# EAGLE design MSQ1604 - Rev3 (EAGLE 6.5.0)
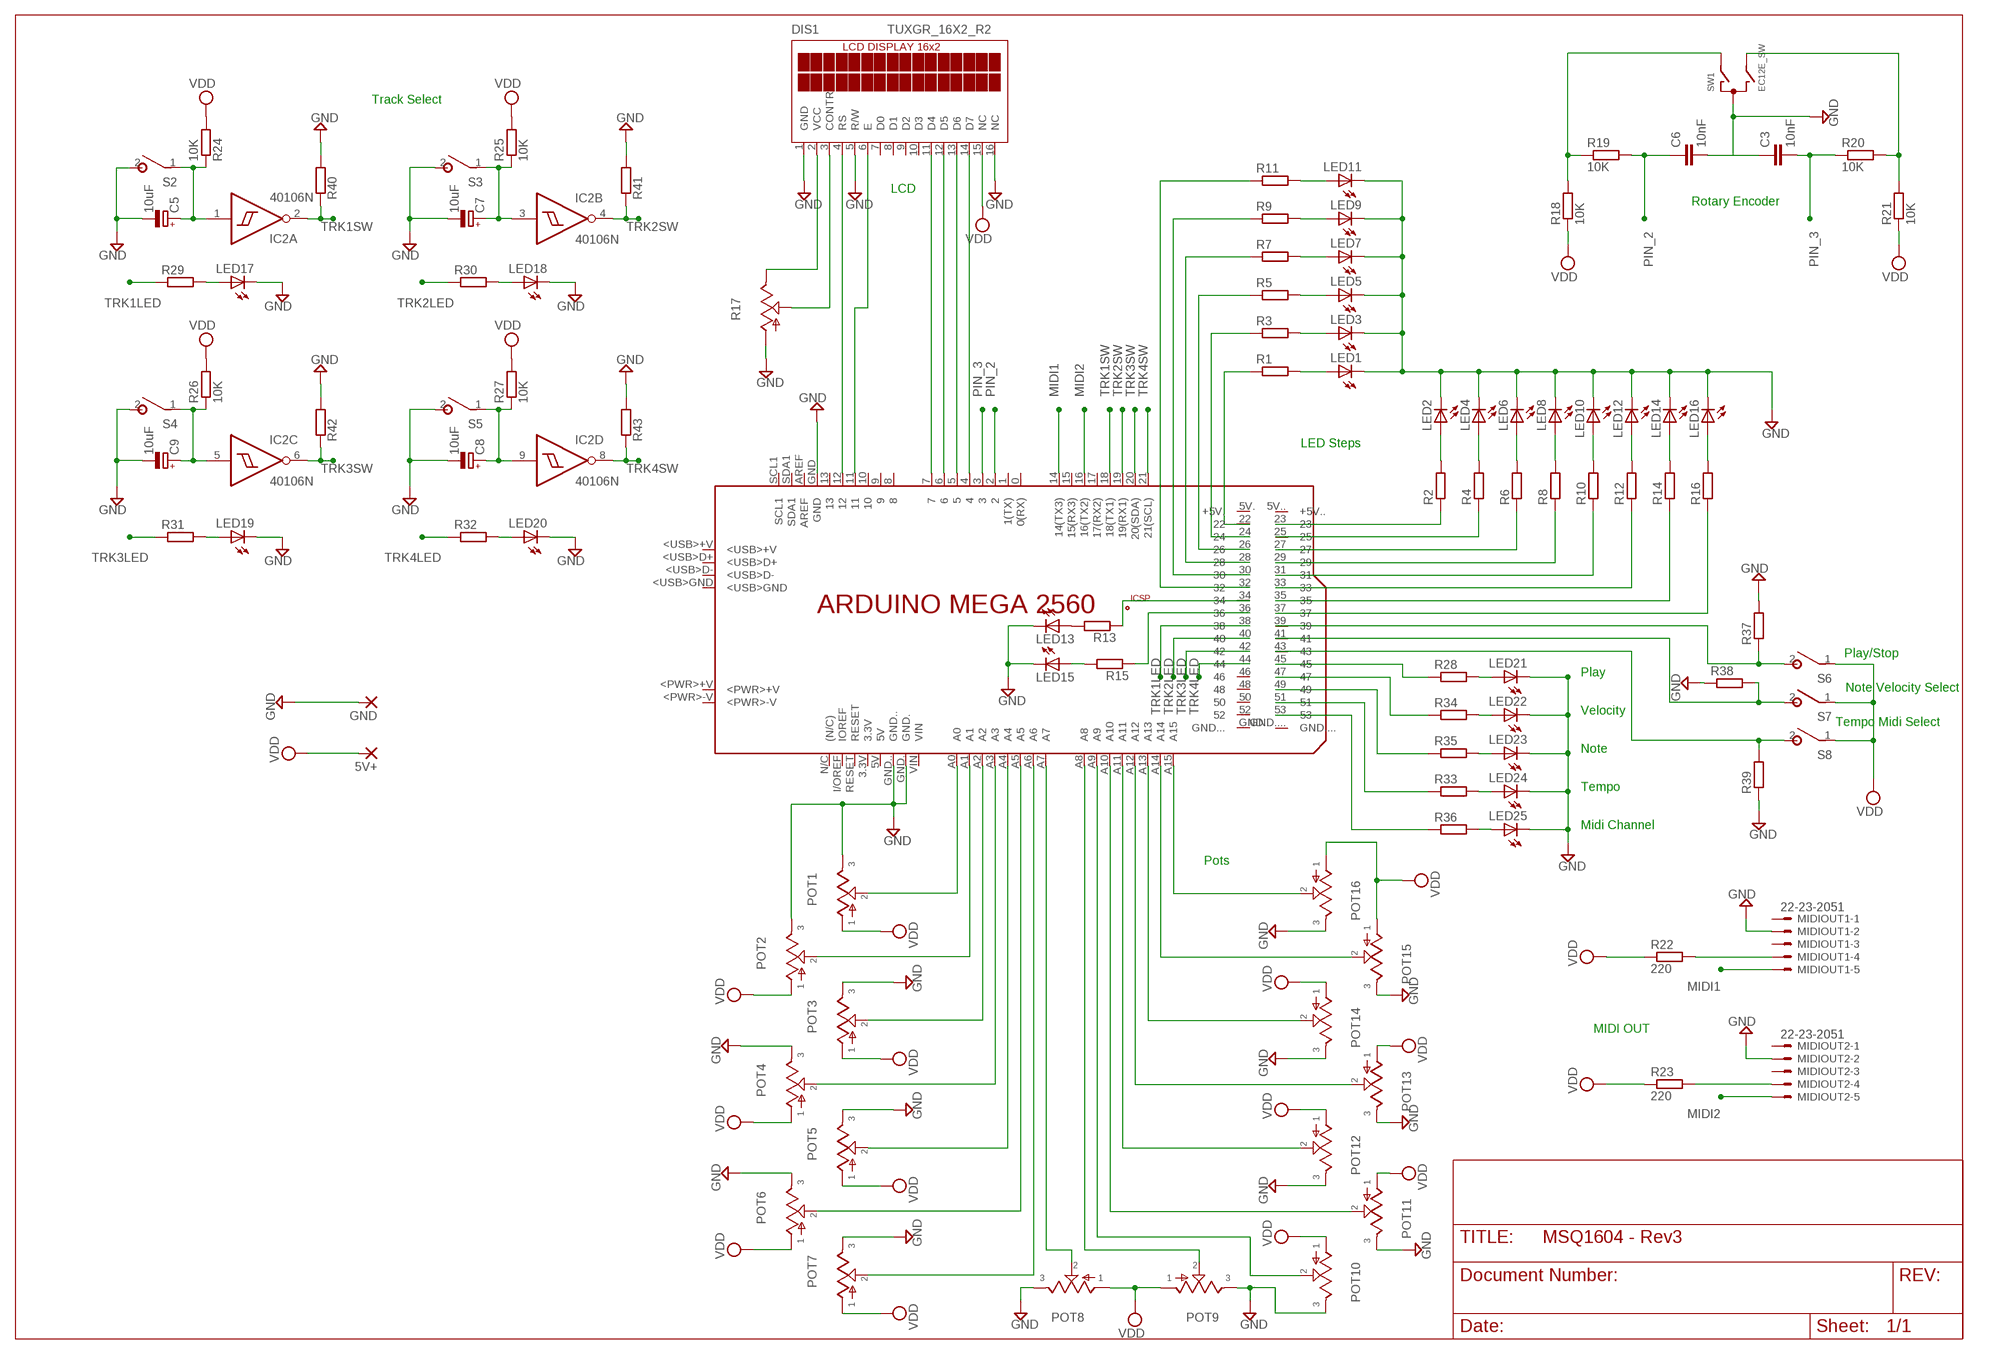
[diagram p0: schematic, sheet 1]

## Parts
5V+  2,54/1,0  [2,54/1,0]
C3  10nF  C-EU050-025X075  [C050-025X075]
C5  10uF  CPOL-EUE2-5  [E2-5]
C6  10nF  C-EU050-025X075  [C050-025X075]
C7  10uF  CPOL-EUE2-5  [E2-5]
C8  10uF  CPOL-EUE2-5  [E2-5]
C9  10uF  CPOL-EUE2-5  [E2-5]
DIS1  TUXGR_16X2_R2  [TUXGR_16X2_R2]
GND  2,54/1,0  [2,54/1,0]
IC2  40106N  [DIL14]
LED1  LEDSQR2X5  [LED2X5]
LED2  LEDSQR2X5  [LED2X5]
LED3  LEDSQR2X5  [LED2X5]
LED4  LEDSQR2X5  [LED2X5]
LED5  LEDSQR2X5  [LED2X5]
LED6  LEDSQR2X5  [LED2X5]
LED7  LEDSQR2X5  [LED2X5]
LED8  LEDSQR2X5  [LED2X5]
LED9  LEDSQR2X5  [LED2X5]
LED10  LEDSQR2X5  [LED2X5]
LED11  LEDSQR2X5  [LED2X5]
LED12  LEDSQR2X5  [LED2X5]
LED13  LEDSQR2X5  [LED2X5]
LED14  LEDSQR2X5  [LED2X5]
LED15  LEDSQR2X5  [LED2X5]
LED16  LEDSQR2X5  [LED2X5]
LED17  LEDSQR2X5  [LED2X5]
LED18  LEDSQR2X5  [LED2X5]
LED19  LEDSQR2X5  [LED2X5]
LED20  LEDSQR2X5  [LED2X5]
LED21  LEDSQR2X5  [LED2X5]
LED22  LEDSQR2X5  [LED2X5]
LED23  LEDSQR2X5  [LED2X5]
LED24  LEDSQR2X5  [LED2X5]
LED25  LEDSQR2X5  [LED2X5]
MIDIOUT1  22-23-2051  [22-23-2051]
MIDIOUT2  22-23-2051  [22-23-2051]
PCB1  ARDUINO_MEGA2560  [ARDUINO_MEGA2560]
POT1  POT  [POT]
POT2  POT  [POT]
POT3  POT  [POT]
POT4  POT  [POT]
POT5  POT  [POT]
POT6  POT  [POT]
POT7  POT  [POT]
POT8  POT  [POT]
POT9  POT  [POT]
POT10  POT  [POT]
POT11  POT  [POT]
POT12  POT  [POT]
POT13  POT  [POT]
POT14  POT  [POT]
POT15  POT  [POT]
POT16  POT  [POT]
R1  R-EU_0204/7  [0204/7]
R2  R-EU_0204/7  [0204/7]
R3  R-EU_0204/7  [0204/7]
R4  R-EU_0204/7  [0204/7]
R5  R-EU_0204/7  [0204/7]
R6  R-EU_0204/7  [0204/7]
R7  R-EU_0204/7  [0204/7]
R8  R-EU_0204/7  [0204/7]
R9  R-EU_0204/7  [0204/7]
R10  R-EU_0204/7  [0204/7]
R11  R-EU_0204/7  [0204/7]
R12  R-EU_0204/7  [0204/7]
R13  R-EU_0204/7  [0204/7]
R14  R-EU_0204/7  [0204/7]
R15  R-EU_0204/7  [0204/7]
R16  R-EU_0204/7  [0204/7]
R17  TRIM_US-CT6  [CT6]
R18  10K  R-EU_0204/7  [0204/7]
R19  10K  R-EU_0204/7  [0204/7]
R20  10K  R-EU_0204/7  [0204/7]
R21  10K  R-EU_0204/7  [0204/7]
R22  220  R-EU_0204/7  [0204/7]
R23  220  R-EU_0204/7  [0204/7]
R24  10K  R-EU_0204/7  [0204/7]
R25  10K  R-EU_0204/7  [0204/7]
R26  10K  R-EU_0204/7  [0204/7]
R27  10K  R-EU_0204/7  [0204/7]
R28  R-EU_0204/7  [0204/7]
R29  R-EU_0204/7  [0204/7]
R30  R-EU_0204/7  [0204/7]
R31  R-EU_0204/7  [0204/7]
R32  R-EU_0204/7  [0204/7]
R33  R-EU_0204/7  [0204/7]
R34  R-EU_0204/7  [0204/7]
R35  R-EU_0204/7  [0204/7]
R36  R-EU_0204/7  [0204/7]
R37  R-EU_0204/7  [0204/7]
R38  R-EU_0204/7  [0204/7]
R39  R-EU_0204/7  [0204/7]
R40  R-EU_0204/7  [0204/7]
R41  R-EU_0204/7  [0204/7]
R42  R-EU_0204/7  [0204/7]
R43  R-EU_0204/7  [0204/7]
S2  SPST  [SPST]
S3  SPST  [SPST]
S4  SPST  [SPST]
S5  SPST  [SPST]
S6  SPST  [SPST]
S7  SPST  [SPST]
S8  SPST  [SPST]
SW1  EC12E_SW  [ALPS_EC12E_SW]

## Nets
GND: C3.1 C5.- C6.2 C7.- C8.- C9.- DIS1.1(GND) DIS1.5(R/W) DIS1.16(NC) GND.1(P) LED1.K(C) LED2.K(C) LED3.K(C) LED4.K(C) LED5.K(C) LED6.K(C) LED7.K(C) LED8.K(C) LED9.K(C) LED10.K(C) LED11.K(C) LED12.K(C) LED13.K(C) LED14.K(C) LED15.K(C) LED16.K(C) LED17.K(C) LED18.K(C) LED19.K(C) LED20.K(C) LED21.K(C) LED22.K(C) LED23.K(C) LED24.K(C) LED25.K(C) MIDIOUT1.2 MIDIOUT2.2 PCB1.GND PCB1.GND. PCB1.GND.. POT1.3 POT2.3 POT3.3 POT4.3 POT5.3 POT6.3 POT7.3 POT8.3 POT9.3 POT10.3 POT11.3 POT12.3 POT13.3 POT14.3 POT15.3 POT16.3 R17.A R37.2 R38.1 R39.1 R40.2 R41.2 R42.2 R43.2 S2.2(S) S3.2(S) S4.2(S) S5.2(S) SW1.C
MIDI1: MIDIOUT1.5 PCB1.14(14(TX3))
MIDI2: MIDIOUT2.5 PCB1.16(16(TX2))
N$1: PCB1.A4 POT5.2
N$2: PCB1.A0 POT1.2
N$4: PCB1.A1 POT2.2
N$5: PCB1.A2 POT3.2
N$6: DIS1.6(E) PCB1.11
N$7: PCB1.A3 POT4.2
N$9: PCB1.A5 POT6.2
N$10: PCB1.A6 POT7.2
N$11: PCB1.A7 POT8.2
N$12: DIS1.12(D5) PCB1.6
N$13: PCB1.A8 POT9.2
N$14: DIS1.4(RS) PCB1.12
N$15: PCB1.A9 POT10.2
N$16: PCB1.A10 POT11.2
N$17: PCB1.A11 POT12.2
N$18: PCB1.A12 POT13.2
N$19: PCB1.A13 POT14.2
N$20: DIS1.14(D7) PCB1.4
N$21: DIS1.13(D6) PCB1.5
N$22: PCB1.A14 POT15.2
N$23: DIS1.11(D4) PCB1.7
N$24: PCB1.22 R1.1
N$25: PCB1.A15 POT16.2
N$26: PCB1.24 R3.1
N$27: PCB1.26 R5.1
N$28: PCB1.28 R7.1
N$29: PCB1.30 R9.1
N$30: PCB1.32 R11.1
N$31: LED15.A R15.2
N$32: PCB1.36 R15.1
N$33: PCB1.23 R2.1
N$34: PCB1.25 R4.1
N$35: PCB1.27 R6.1
N$36: PCB1.29 R8.1
N$37: PCB1.31 R10.1
N$38: PCB1.33 R12.1
N$39: PCB1.35 R14.1
N$40: PCB1.37 R16.1
N$42: LED16.A R16.2
N$43: LED14.A R14.2
N$44: LED12.A R12.2
N$45: LED10.A R10.2
N$46: LED8.A R8.2
N$47: LED6.A R6.2
N$48: LED4.A R4.2
N$49: LED2.A R2.2
N$50: C5.+ IC2.1(A:I) R24.1 S2.1(P)
N$51: LED19.A R31.2
N$52: LED1.A R1.2
N$53: LED11.A R11.2
N$54: LED9.A R9.2
N$55: LED7.A R7.2
N$56: LED5.A R5.2
N$57: LED3.A R3.2
N$58: PCB1.34 R13.1
N$59: LED13.A R13.2
N$60: C9.+ IC2.5(C:I) R26.1 S4.1(P)
N$61: C8.+ IC2.9(D:I) R27.1 S5.1(P)
N$62: LED20.A R32.2
N$63: C7.+ IC2.3(B:I) R25.1 S3.1(P)
N$64: LED18.A R30.2
N$65: PCB1.41 R38.2 S7.2(S)
N$66: LED17.A R29.2
N$67: PCB1.39 R37.1 S6.2(S)
N$68: DIS1.2(VCC) R17.E
N$69: PCB1.45 R28.1
N$70: DIS1.3(CONTR) R17.S
N$71: PCB1.43 R39.2 S8.2(S)
N$72: R18.2 R19.1 SW1.A
N$73: MIDIOUT1.4 R22.2
N$74: R20.2 R21.2 SW1.B
N$75: PCB1.49 R35.1
N$76: LED21.A R28.2
N$77: MIDIOUT2.4 R23.2
N$78: LED22.A R34.2
N$79: LED23.A R35.2
N$80: PCB1.47 R34.1
N$81: LED25.A R36.2
N$82: LED24.A R33.2
N$83: PCB1.53 R36.1
N$85: PCB1.51 R33.1
PIN_2: C6.1 PCB1.2 R19.2
PIN_3: C3.2 PCB1.3 R20.1
TRK1LED: PCB1.38 R29.1
TRK1SW: IC2.2(A:O) PCB1.18(18(TX1)) R40.1
TRK2LED: PCB1.40 R30.1
TRK2SW: IC2.4(B:O) PCB1.19(19(RX1)) R41.1
TRK3LED: PCB1.42 R31.1
TRK3SW: IC2.6(C:O) PCB1.20(20(SDA)) R42.1
TRK4LED: PCB1.44 R32.1
TRK4SW: IC2.8(D:O) PCB1.21(21(SCL)) R43.1
VDD: 5V+.1(P) DIS1.15(NC) POT1.1 POT2.1 POT3.1 POT4.1 POT5.1 POT6.1 POT7.1 POT8.1 POT9.1 POT10.1 POT11.1 POT12.1 POT13.1 POT14.1 POT15.1 POT16.1 R18.1 R21.1 R22.1 R23.1 R24.2 R25.2 R26.2 R27.2 S6.1(P) S7.1(P) S8.1(P)
Unconnected: DIS1.7(D0) DIS1.8(D1) DIS1.9(D2) DIS1.10(D3) IC2.10(E:O) IC2.11(E:I) IC2.12(F:O) IC2.13(F:I) MIDIOUT1.1 MIDIOUT1.3 MIDIOUT2.1 MIDIOUT2.3 PCB1.0(0(RX)) PCB1.1(1(TX)) PCB1.3.3V PCB1.5V PCB1.5V.(+5V.) PCB1.5V..(+5V..) PCB1.8 PCB1.9 PCB1.10 PCB1.13 PCB1.15(15(RX3)) PCB1.17(17(RX2)) PCB1.46 PCB1.48 PCB1.50 PCB1.52 PCB1.+5V_ PCB1.<PWR>+V PCB1.<PWR>-V PCB1.<USB>+V PCB1.<USB>D+ PCB1.<USB>D- PCB1.<USB>GND PCB1.AREF PCB1.GND... PCB1.GND.... PCB1.GND__ PCB1.I/OREF(IOREF) PCB1.MISO PCB1.MOSI PCB1.N/C((N/C)) PCB1.RESET PCB1.RESET. PCB1.SCK PCB1.SCL1 PCB1.SDA1 PCB1.VIN SW1.D SW1.E SW1.GND1(G) SW1.GND2(G)

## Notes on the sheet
- Track Select
- LCD
- Rotary Encoder
- LED Steps
- Play/Stop
- Play
- Note Velocity Select
- Velocity
- Tempo Midi Select
- Note
- Tempo
- Midi Channel
- Pots
- MIDI OUT

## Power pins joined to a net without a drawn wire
VDD: IC2.14(P:VDD)
VSS: IC2.7(P:VSS)

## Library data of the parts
5V+ GND = wirepad:2,54/1,0: THROUGH-HOLE PAD
C3 C6 = resistor:C-EU: CAPACITOR, European symbol
C5 C7-C9 = resistor:CPOL-EU: POLARIZED CAPACITOR, European symbol
DIS1 = display-lcd:TUXGR_16X2_R2: Tuxgraphics LCD display 16x2 characters reflective, without background light Source: tuxgr_12x2_r2.pdf; OC_FARNELL: unknown; OC_NEWARK: unknown
IC2 = 40xx:40106: Hex SCHMITT TRIGGER
LED1-LED25 = led:LED: LED
MIDIOUT1 MIDIOUT2 = con-molex:22-23-2051: .100" (2.54mm) Center Header - 5 Pin; MF: MOLEX; MPN: 22-23-2051; OC_FARNELL: 1462952; OC_NEWARK: 38C9178
PCB1 = E14_Arduino_revB:ARDUINO_MEGA2560: Device for representing an Arduino Mega 2560 board with a footprint in an EAGLE design. Created by Dave Young for Element14. More EAGLE documentation at: http://www.element14.com/community/community/knode/cadsoft_eagle
POT1-POT16 = gm-pots:POT: Potentiometers the arrow indicates the clockwise motion of th wiper (lug 2) fully counter clockwise there is no resistance between lugs 1 and 2 fully clockwise the resistance between lugs 1 and 2 is the value of the pot
R1-R16 R18-R43 = resistor:R-EU_: RESISTOR, European symbol
R17 = pot:TRIM_US-: POTENTIOMETER
S2-S8 = gm-switches:SPST
SW1 = switch-alps:EC12E_SW: ALPS rotary Encoder EC12E series with switch; MPN: EC12E2424407; OC_FARNELL: 1520813; OC_NEWARK: 74M1068

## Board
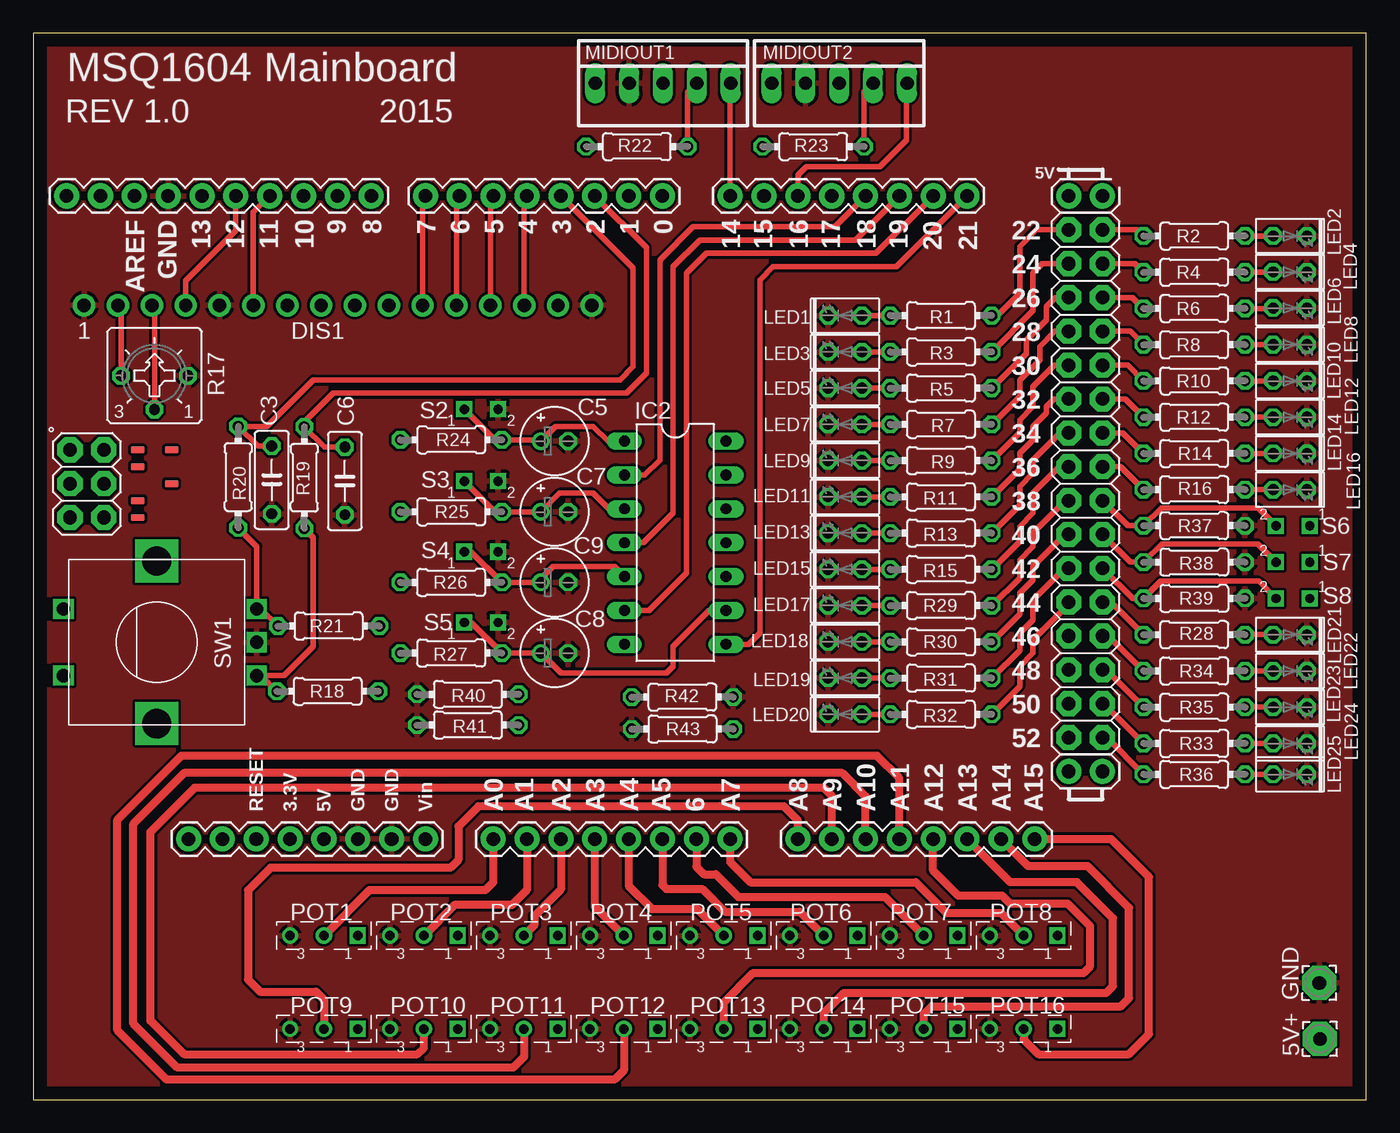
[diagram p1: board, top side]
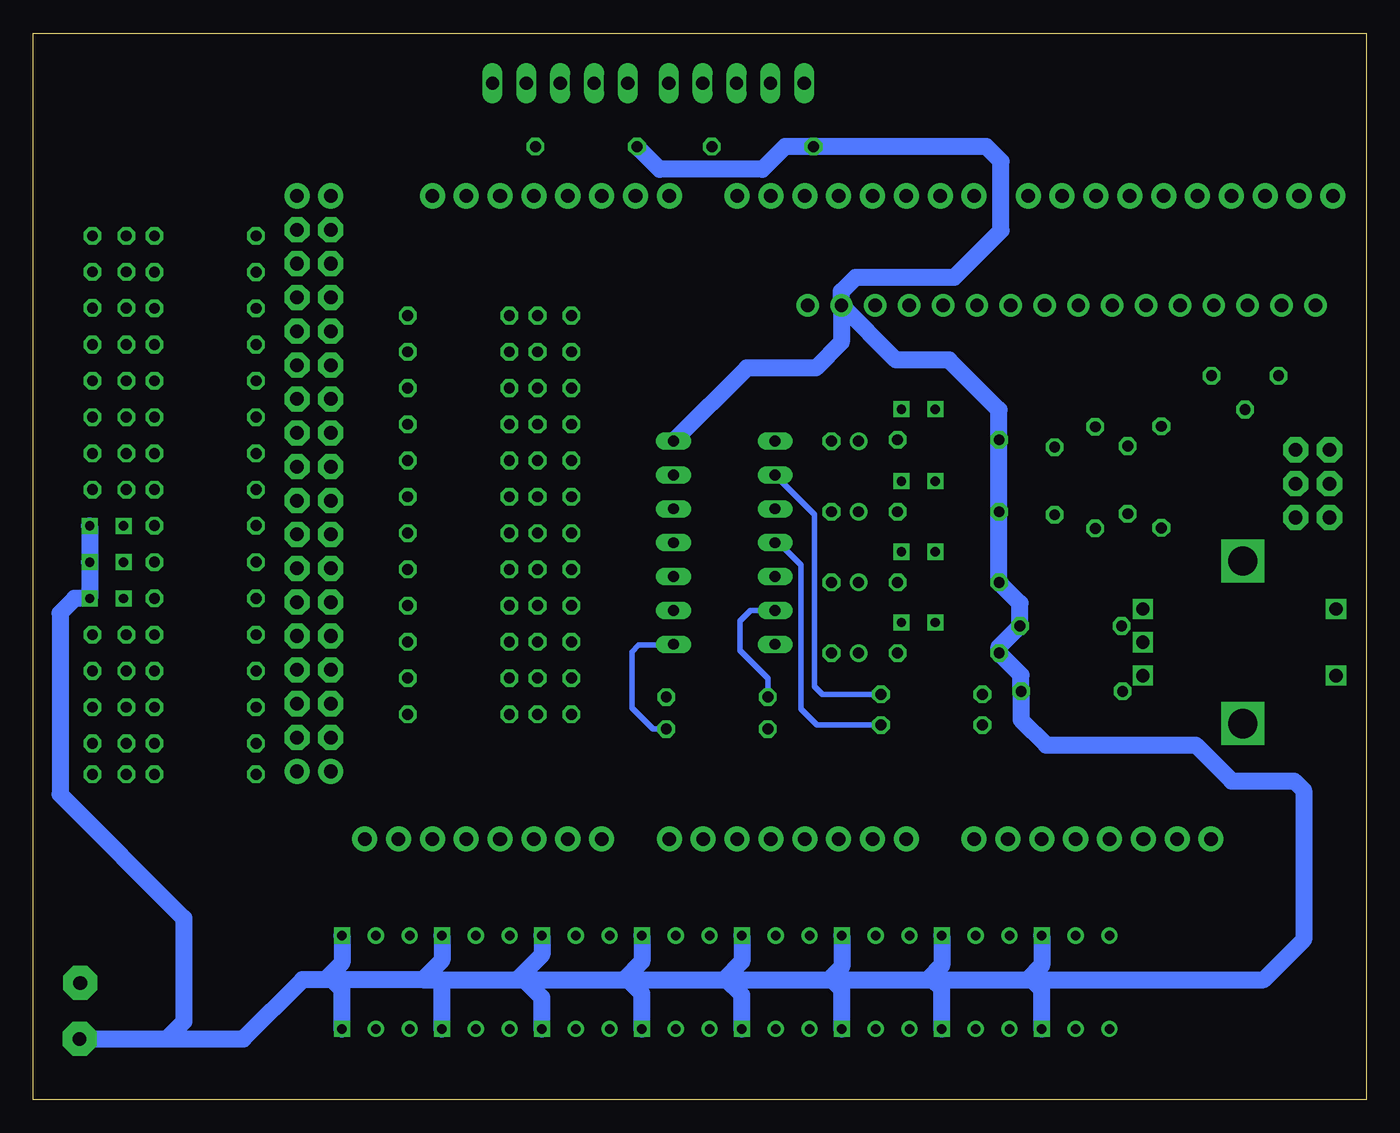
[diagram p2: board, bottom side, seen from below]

Size 100 x 80 mm. Coordinates in mm from the lower left corner, seen from the top.
Outline: 0,0 100,0 100,80 0,80 0,0
Copper layers (1*16): Top 0.035mm / dielectric 1.5mm / Bottom 0.035mm
Design rules "default": minimum track width 10mil, minimum drill 24mil, track to track 8mil, track to pad 8mil, pad to pad 8mil, via to via 8mil, smd to smd 8mil, copper to edge 40mil, drill to drill 8mil, minimum pad ring 10mil, minimum via ring 8mil, stop-mask expansion 4mil, vias tented up to drill 0mil, thermal gap 10mil

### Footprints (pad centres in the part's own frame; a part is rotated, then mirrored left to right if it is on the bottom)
2,54/1,0 = drill 1.016 pad 2.54 octagon: 1 0,0
C050-025X075 = drill 0.813 octagon: 1 -2.54,0; 2 2.54,0
E2-5 = drill 0.813 pad 1.27: + -1.016,0 | drill 0.813 pad 1.27 octagon: - 1.016,0
TUXGR_16X2_R2 = drill 1 pad 1.676: 1 1.02,1.53; 2 3.56,1.53; 3 6.1,1.53; 4 8.64,1.53; 5 11.18,1.53; 6 13.72,1.53; 7 16.26,1.53; 8 18.8,1.53; 9 21.34,1.53; 10 23.88,1.53; 11 26.42,1.53; 12 28.96,1.53; 13 31.5,1.53; 14 34.04,1.53; 15 36.58,1.53; 16 39.12,1.53
DIL14 = drill 0.813 long: 1 -7.62,-3.81; 2 -5.08,-3.81; 3 -2.54,-3.81; 4 0,-3.81; 5 2.54,-3.81; 6 5.08,-3.81; 7 7.62,-3.81; 8 7.62,3.81; 9 5.08,3.81; 10 2.54,3.81; 11 0,3.81; 12 -2.54,3.81; 13 -5.08,3.81; 14 -7.62,3.81
LED2X5 = drill 0.813 octagon: A -1.27,0; K 1.27,0
22-23-2051 = drill 1 long: 1 -5.08,0; 2 -2.54,0; 3 0,0; 4 2.54,0; 5 5.08,0
ARDUINO_MEGA2560 = drill 1.016 pad 1.88: 0 63.5,50.8; 1 60.96,50.8; 2 58.42,50.8; 3 55.88,50.8; 3.3V 35.56,2.54; 4 53.34,50.8; 5 50.8,50.8; 5V 38.1,2.54; 5V. 93.98,50.8; 5V.. 96.52,50.8; 6 48.26,50.8; 7 45.72,50.8; 8 41.656,50.8; 9 39.116,50.8; 10 36.576,50.8; 11 34.036,50.8; 12 31.496,50.8; 13 28.956,50.8; 14 68.58,50.8; 15 71.12,50.8; 16 73.66,50.8; 17 76.2,50.8; 18 78.74,50.8; 19 81.28,50.8; 20 83.82,50.8; 21 86.36,50.8; A0 50.8,2.54; A1 53.34,2.54; A2 55.88,2.54; A3 58.42,2.54; A4 60.96,2.54; A5 63.5,2.54; A6 66.04,2.54; A7 68.58,2.54; A8 73.66,2.54; A9 76.2,2.54; A10 78.74,2.54; A11 81.28,2.54; A12 83.82,2.54; A13 86.36,2.54; A14 88.9,2.54; A15 91.44,2.54; AREF 23.876,50.8; GND 26.416,50.8; GND. 43.18,2.54; GND.. 40.64,2.54; GND... 93.98,7.62; GND.... 96.52,7.62; I/OREF 30.48,2.54; N/C 27.94,2.54; RESET 33.02,2.54; SCL1 18.796,50.8; SDA1 21.336,50.8; VIN 45.72,2.54 | drill 1.016 pad 1.88 octagon: 22 93.98,48.26; 23 96.52,48.26; 24 93.98,45.72; 25 96.52,45.72; 26 93.98,43.18; 27 96.52,43.18; 28 93.98,40.64; 29 96.52,40.64; 30 93.98,38.1; 31 96.52,38.1; 32 93.98,35.56; 33 96.52,35.56; 34 93.98,33.02; 35 96.52,33.02; 36 93.98,30.48; 37 96.52,30.48; 38 93.98,27.94; 39 96.52,27.94; 40 93.98,25.4; 41 96.52,25.4; 42 93.98,22.86; 43 96.52,22.86; 44 93.98,20.32; 45 96.52,20.32; 46 93.98,17.78; 47 96.52,17.78; 48 93.98,15.24; 49 96.52,15.24; 50 93.98,12.7; 51 96.52,12.7; 52 93.98,10.16; 53 96.52,10.16; +5V_ 21.59,31.75; GND__ 21.59,26.67; MISO 19.05,31.75; MOSI 21.59,29.21; RESET. 19.05,26.67; SCK 19.05,29.21 | smd 1.016 x 0.508: <PWR>+V 26.67,31.75; <PWR>-V 26.67,29.21; <USB>+V 24.13,31.75; <USB>D+ 24.13,30.48; <USB>D- 24.13,27.94; <USB>GND 24.13,26.67
POT = drill 0.7 square: 1 2.54,0 | drill 0.7: 2 0,0; 3 -2.54,0
0204/7 = drill 0.813 octagon: 1 -3.81,0; 2 3.81,0
CT6 = drill 0.813 octagon: A 2.515,0; E -2.515,0; S 0,-2.54
SPST = drill 0.7 square: 1 -1.27,0; 2 1.27,0
ALPS_EC12E_SW = drill 1 square: A -2.5,-7.5; B 2.5,-7.5; C 0,-7.5; D -2.5,7; E 2.5,7 | drill 2.2 square: GND1 -6.1,0; GND2 6.1,0

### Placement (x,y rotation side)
5V+  96.53,4.55 90 top
C3  17.89,46.49 90 top
C5  39.1,49.4 0 top
C6  23.37,46.41 270 top
C7  39.1,44.1 0 top
C8  39.1,33.5 0 top
C9  39.1,38.8 0 top
DIS1  2.79,58.07 0 top
GND  96.48,8.75 90 top
IC2  48.16,41.78 270 top
LED1  60.9,58.82 180 top
LED2  94.29,64.8 0 top
LED3  60.9,56.1 180 top
LED4  94.29,62.1 0 top
LED5  60.9,53.38 180 top
LED6  94.29,59.39 0 top
LED7  60.9,50.66 180 top
LED8  94.29,56.64 0 top
LED9  60.9,47.94 180 top
LED10  94.29,53.92 0 top
LED11  60.9,45.22 180 top
LED12  94.29,51.2 0 top
LED13  60.9,42.5 180 top
LED14  94.29,48.48 0 top
LED15  60.9,39.78 180 top
LED16  94.29,45.76 0 top
LED17  60.9,37.06 180 top
LED18  60.9,34.34 180 top
LED19  60.9,31.62 180 top
LED20  60.9,28.9 180 top
LED21  94.29,34.88 0 top
LED22  94.29,32.16 0 top
LED23  94.29,29.44 0 top
LED24  94.29,26.72 0 top
LED25  94.29,24.4 0 top
MIDIOUT1  47.24,76.26 0 top
MIDIOUT2  60.47,76.26 0 top
PCB1  -16.3,17 0 top
POT1  21.8,12.3 0 top
POT2  29.3,12.3 0 top
POT3  36.8,12.3 0 top
POT4  44.3,12.3 0 top
POT5  51.8,12.3 0 top
POT6  59.3,12.3 0 top
POT7  66.8,12.3 0 top
POT8  74.3,12.3 0 top
POT9  21.8,5.3 0 top
POT10  29.3,5.3 0 top
POT11  36.8,5.3 0 top
POT12  44.3,5.3 0 top
POT13  51.8,5.3 0 top
POT14  59.3,5.3 0 top
POT15  66.8,5.3 0 top
POT16  74.3,5.3 0 top
R1  68.1,58.82 180 top
R2  87.1,64.8 0 top
R3  68.1,56.1 180 top
R4  87.1,62.08 0 top
R5  68.1,53.38 180 top
R6  87.1,59.36 0 top
R7  68.1,50.66 180 top
R8  87.1,56.64 0 top
R9  68.1,47.94 180 top
R10  87.1,53.92 0 top
R11  68.1,45.22 180 top
R12  87.1,51.2 0 top
R13  68.1,42.5 180 top
R14  87.1,48.48 0 top
R15  68.1,39.78 180 top
R16  87.1,45.76 0 top
R17  9.09,54.31 0 top
R18  22.08,30.63 180 top
R19  20.33,46.66 90 top
R20  15.37,46.7 270 top
R21  22.16,35.53 180 top
R22  45.28,71.5 0 top
R23  58.52,71.5 0 top
R24  31.35,49.5 180 top
R25  31.35,44.1 180 top
R26  31.35,38.8 180 top
R27  31.35,33.5 180 top
R28  87.1,34.88 0 top
R29  68.1,37.06 180 top
R30  68.1,34.34 180 top
R31  68.1,31.62 180 top
R32  68.1,28.9 180 top
R33  87.1,26.72 0 top
R34  87.1,32.16 0 top
R35  87.1,29.44 0 top
R36  87.1,24.4 0 top
R37  87.1,43.06 0 top
R38  87.1,40.32 180 top
R39  87.1,37.6 180 top
R40  32.6,30.4 180 top
R41  32.6,28.1 180 top
R42  48.7,30.2 0 top
R43  48.7,27.8 180 top
S2  33.6,51.8 0 top
S3  33.6,46.4 0 top
S4  33.6,41.1 0 top
S5  33.6,35.8 0 top
S6  94.5,43.04 180 top
S7  94.5,40.32 180 top
S8  94.5,37.6 180 top
SW1  9.26,34.31 90 top

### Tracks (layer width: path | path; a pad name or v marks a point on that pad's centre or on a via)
GND
  pour Top: -10,90 110,90 110,-10 -10,-10
MIDI1
  Top 0.406: PCB1.14 52.28,76.22 MIDIOUT1.5
MIDI2
  Top 0.406: PCB1.16 57.36,69.36 58,70 63.5,70 65.5,72 65.5,76.21 MIDIOUT2.5
N$1
  Top 0.61: PCB1.A4 44.66,16.04 46.4,14.3 49.8,14.3 POT5.2
N$2
  Top 0.61: PCB1.A0 34.5,16.3 33.9,15.7 25.2,15.7 POT1.2
N$4
  Top 0.61: PCB1.A1 37.04,15.74 35.9,14.6 31.6,14.6 POT2.2
N$5
  Top 0.61: PCB1.A2 39.58,15.78 37.6,13.8 37.6,13.1 POT3.2
N$6
  Top 0.406: DIS1.6 16.51,66.57 PCB1.11
N$7
  Top 0.61: PCB1.A3 42.12,14.48 POT4.2
N$9
  Top 0.61: PCB1.A5 47.2,16.1 47.5,15.8 50.2,15.8 51.9,14.1 57.5,14.1 POT6.2
N$10
  Top 0.61: PCB1.A6 49.74,17.46 50.3,16.9 51.2,16.9 52.9,15.2 63.9,15.2 POT7.2
N$11
  Top 0.61: PCB1.A7 52.28,17.82 53.8,16.3 66.2,16.3 68.5,14 72.6,14 POT8.2
N$12
  Top 0.406: DIS1.12 31.75,67.59 PCB1.6
N$13
  Top 0.61: PCB1.A8 57.36,20.94 56.3,22 33.4,22 31.9,20.5 31.9,18 31.3,17.4 17.8,17.4 16.1,15.7 16.1,9 17,8.1 21.2,8.1 21.8,7.5 POT9.2
N$14
  Top 0.406: DIS1.4 11.43,61.43 15.2,65.2 PCB1.12
N$15
  Top 0.61: PCB1.A9 59.9,22.8 59.3,23.4 12.1,23.4 8.8,20.1 8.8,5.9 11.3,3.4 28.8,3.4 29.3,3.9 POT10.2
N$16
  Top 0.61: PCB1.A10 62.44,22.76 60.7,24.5 11.3,24.5 7.5,20.7 7.5,5.7 10.8,2.4 36,2.4 36.8,3.2 POT11.2
N$17
  Top 0.61: PCB1.A11 64.98,24.12 63.3,25.8 11.1,25.8 6.3,21 6.3,5.2 10,1.5 43.6,1.5 44.3,2.2 POT12.2
N$18
  Top 0.61: POT13.2 51.8,7.3 54,9.5 78.8,9.5 79.3,10 79.3,13 77.6,14.7 73.3,14.7 72.7,15.3 69.4,15.3 67.5,17.2 67.5,19.52 PCB1.A12
N$19
  Top 0.61: POT14.2 59.3,6.5 60.8,8 80.5,8 81,8.5 81,13.6 78.3,16.3 73.3,16.3 PCB1.A13
N$20
  Top 0.406: DIS1.14 36.83,67.59 PCB1.4
N$21
  Top 0.406: DIS1.13 34.29,67.59 PCB1.5
N$22
  Top 0.61: PCB1.A14 74.64,17.5 79.1,17.5 82.2,14.4 82.2,7.6 81.6,7 67.4,7 66.8,6.4 POT15.2
N$23
  Top 0.406: DIS1.11 29.21,67.59 PCB1.7
N$24
  Top 0.406: R1.1 72.32,58.82 74,60.5 74,64 75.26,65.26 PCB1.22
N$25
  Top 0.61: PCB1.A15 80.86,19.54 83.7,16.7 83.7,4.9 82.2,3.4 75.4,3.4 74.3,4.5 POT16.2
N$26
  Top 0.406: PCB1.24 75.72,62.72 75,62 75,59.19 R3.1
N$27
  Top 0.406: PCB1.26 76.68,60.18 76,59.5 76,58.5 74.5,57 74.5,55.97 R5.1
N$28
  Top 0.406: PCB1.28 76.64,57.64 75.5,56.5 75.5,55.5 74,54 74,52.75 R7.1
N$29
  Top 0.406: PCB1.30 76.6,55.1 75,53.5 75,52 74,51 74,50.03 R9.1
N$30
  Top 0.406: PCB1.32 76.56,52.56 76,52 76,51.5 75,50.5 75,49.5 74,48.5 74,47.31 R11.1
N$31
  Top 0.406: LED15.A R15.2
N$32
  Top 0.406: PCB1.36 76.98,47.48 75,45.5 75,44 74,43 74,41.87 R15.1
N$33
  Top 0.406: PCB1.23 82.83,65.26 R2.1
N$34
  Top 0.406: PCB1.25 82.65,62.72 R4.1
N$35
  Top 0.406: PCB1.27 82.47,60.18 R6.1
N$36
  Top 0.406: PCB1.29 82.29,57.64 R8.1
N$37
  Top 0.406: PCB1.31 82.11,55.1 R10.1
N$38
  Top 0.406: PCB1.33 81.93,52.56 R12.1
N$39
  Top 0.406: PCB1.35 81.75,50.02 R14.1
N$40
  Top 0.406: PCB1.37 81.57,47.48 R16.1
N$42
  Top 0.406: R16.2 LED16.A
N$43
  Top 0.406: R14.2 LED14.A
N$44
  Top 0.406: R12.2 LED12.A
N$45
  Top 0.406: R10.2 LED10.A
N$46
  Top 0.406: R8.2 LED8.A
N$47
  Top 0.406: R6.2 92.99,59.36 LED6.A
N$48
  Top 0.406: R4.2 93,62.08 LED4.A
N$49
  Top 0.406: R2.2 LED2.A
N$50
  Top 0.406: S2.1 34.63,49.5 R24.1 37.98,49.5 C5.+ 39.18,50.5 42,50.5 43.1,49.4 IC2.1
N$51
  Top 0.406: LED19.A R31.2
N$52
  Top 0.406: LED1.A R1.2
N$53
  Top 0.406: LED11.A R11.2
N$54
  Top 0.406: LED9.A R9.2
N$55
  Top 0.406: LED7.A R7.2
N$56
  Top 0.406: LED5.A R5.2
N$57
  Top 0.406: LED3.A R3.2
N$58
  Top 0.406: PCB1.34 77.02,50.02 75,48 75,47 74,46 74,44.59 R13.1
N$59
  Top 0.406: LED13.A R13.2
N$60
  Top 0.406: S4.1 32.86,41.1 R26.1 C9.+ 38.08,39.08 39,40 43.59,40 IC2.5
N$61
  Top 0.406: S5.1 32.86,35.8 R27.1 C8.+ 39.58,32 47.5,32 48,32.5 48,34 50.7,36.7 IC2.9
N$62
  Top 0.406: LED20.A R32.2
N$63
  Top 0.406: IC2.3 43.18,44.32 42,45.5 39.48,45.5 C7.+ R25.1 34.63,44.1 S3.1
N$64
  Top 0.406: LED18.A R30.2
N$65
  Top 0.406: PCB1.41 82.3,40.32 R38.2 84.67,41.7 91.85,41.7 S7.2
N$66
  Top 0.406: LED17.A R29.2
N$67
  Top 0.406: PCB1.39 82.1,43.06 R37.1 84.63,44.4 91.9,44.4 93.23,43.07 S6.2
N$68
  Top 0.406: R17.E 6.58,59.38 DIS1.2
N$69
  Top 0.406: PCB1.45 80.85,37.32 R28.1
N$70
  Top 0.406: R17.S 9.09,59.4 DIS1.3
N$71
  Top 0.406: PCB1.43 82.48,37.6 R39.2 84.59,38.9 91.93,38.9 S8.2
N$72
  Top 0.406: R18.2 17.09,31.81 SW1.A 18.81,31.81 21,34 21,42.18 R19.1
N$73
  Top 0.406: R22.2 49.09,75.57 MIDIOUT1.4
N$74
  Top 0.406: R21.2 17.07,36.81 SW1.B 16.76,41.5 R20.2
N$75
  Top 0.406: PCB1.49 80.49,32.24 R35.1
N$76
  Top 0.406: R28.2 LED21.A
N$77
  Top 0.406: R23.2 62.33,75.58 MIDIOUT2.4
N$78
  Top 0.406: R34.2 LED22.A
N$79
  Top 0.406: R35.2 LED23.A
N$80
  Top 0.406: PCB1.47 80.67,34.78 R34.1
N$81
  Top 0.406: R36.2 LED25.A
N$82
  Top 0.406: R33.2 LED24.A
N$83
  Top 0.406: PCB1.53 80.53,27.16 R36.1
N$85
  Top 0.406: PCB1.51 80.31,29.7 R33.1
PIN_2
  Top 0.406: C6.1 21.85,48.95 R19.2 20.33,50.83 22.5,53 44.5,53 46,54.5 46,63.92 PCB1.2
PIN_3
  Top 0.406: C3.2 16.85,49.03 R20.1 17.51,50.51 21,54 44,54 45,55 45,62.38 PCB1.3
TRK1LED
  Top 0.406: PCB1.38 77.44,44.94 75,42.5 75,41.5 74,40.5 74,39.15 R29.1
TRK1SW
  Top 0.406: IC2.2 45.86,46.86 47,48 47,63 49.5,65.5 60.14,65.5 PCB1.18
  Bottom 0.406: R40.1 40.8,30.4 41.4,31 41.4,43.91 IC2.2
TRK2LED
  Top 0.406: PCB1.40 77.4,42.4 75,40 75,39 74,38 74,36.43 R30.1
TRK2SW
  Top 0.406: IC2.4 45.78,41.78 48,44 48,62.5 50,64.5 61.68,64.5 PCB1.19
  Bottom 0.406: IC2.4 44.08,41.78 42.4,40.1 42.4,29.3 41.2,28.1 R41.1
TRK3LED
  Top 0.406: PCB1.42 77.36,39.86 75,37.5 75,36 74,35 74,33.71 R31.1
TRK3SW
  Top 0.406: IC2.6 46.2,36.7 49,39.5 49,62 50.5,63.5 63.22,63.5 PCB1.20
  Bottom 0.406: R42.1 44.89,31.59 47,33.7 47,35.9 46.2,36.7 IC2.6
TRK4LED
  Top 0.406: PCB1.44 77.68,37.18 75,34.5 75,33.5 74,32.5 74,30.99 R32.1
TRK4SW
  Top 0.406: IC2.8 53.66,34.16 54.5,35 54.5,61.5 55.5,62.5 64.76,62.5 PCB1.21
  Bottom 0.406: R43.1 53.5,27.8 55.1,29.4 55.1,33.6 54.6,34.1 52.03,34.1 IC2.8
VDD
  Bottom 1.27: DIS1.15 35.27,55.5 31.3,55.5 27.54,51.74 R24.2 R25.2 R26.2 25.97,37.23 R21.1 27.54,33.96 R27.2 25.89,31.85 R18.1 25.89,28.49 24,26.6 12.8,26.6 10.1,23.9 5.4,23.9 4.7,23.2 4.7,12 7.7,9 25.1,9 | DIS1.15 39.37,60.63 38.3,61.7 30.9,61.7 27.4,65.2 27.4,70.4 28.5,71.5 R22.1 43.6,71.5 45.3,69.8 53.01,69.8 R23.1 | DIS1.15 39.37,56.83 41.3,54.9 46.47,54.9 IC2.14 | 5V+.1 90,4.55 | 90,4.55 84.25,4.55 79.8,9 78.1,9 | 70.8,9 69.6,9 | 69.6,9 63.7,9 | 63.7,9 63.2,9 | 63.2,9 55.7,9 | 55.7,9 55.4,9 | 55.4,9 48.2,9 | 48.2,9 48,9 | 48,9 40.3,9 | 40.3,9 40.1,9 | 40.1,9 32.9,9 | 32.9,9 32.5,9 | 32.5,9 25.4,9 | 25.4,9 25.1,9 | 69.6,9 69.34,8.74 POT15.1 | POT7.1 69.34,10.46 70.8,9 | 70.8,9 77.6,9 | 77.6,9 78.1,9 | POT8.1 76.84,10.26 78.1,9 | POT16.1 76.84,8.24 77.6,9 | POT6.1 61.84,10.86 63.7,9 | POT14.1 61.84,7.64 63.2,9 | POT5.1 54.34,10.36 55.7,9 | POT13.1 54.34,7.94 55.4,9 | POT4.1 46.84,10.36 48.2,9 | POT12.1 46.84,7.84 48,9 | POT3.1 39.34,9.96 40.3,9 | POT11.1 39.34,8.24 40.1,9 | POT2.1 31.84,10.06 32.9,9 | POT10.1 31.84,8.34 32.5,9 | POT1.1 24.34,10.06 25.4,9 | POT9.1 24.34,8.24 25.1,9 | S6.1 S7.1 S8.1 96.9,37.6 98,36.5 98,22.9 88.7,13.6 88.7,5.85 90,4.55

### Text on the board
tNames: MSQ1604 Mainboard | REV 1.0 2015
